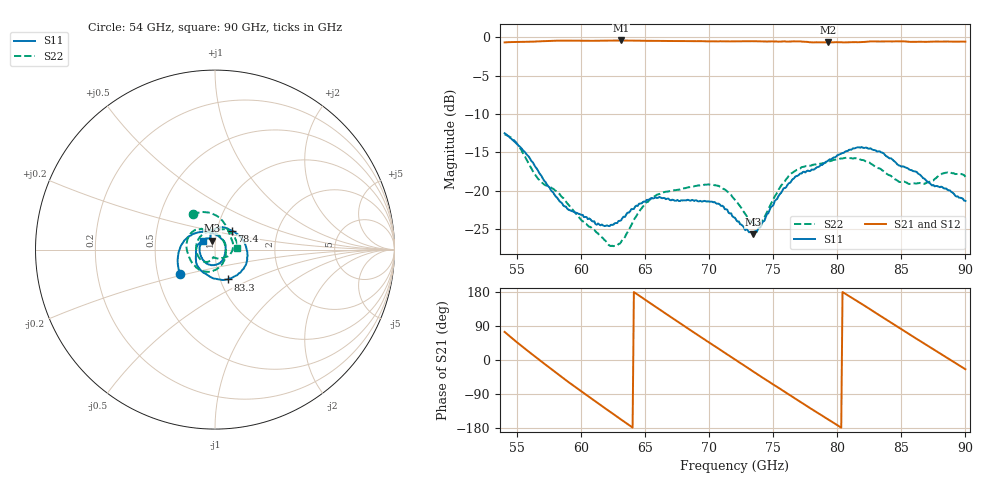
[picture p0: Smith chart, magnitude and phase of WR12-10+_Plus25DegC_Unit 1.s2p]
!Mini-Circuits Laboratory
!S-Parameters
!Model: WR12-10+
!Run / Lot / Date Code: Y97271 / QN2608234 / 2608
!Fixture: N/A, Pressing Arm: N/A
!Network Analyzer: PNA-X N5242B - 423 4 ports (COM/DCOM);  Serial number: 76642
!Date: 3/10/2026 at 2:21:42 PM
!No.: Unit# 1
!Tested with:
# Hz  S  dB  R  50
!Frequency  S11 dB  S11 Deg  S21 dB  S21 Deg  S12 dB  S12 Deg  S22 dB  S22 Deg
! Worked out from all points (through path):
!   352 points, 54 GHz to 90 GHz, reference 50 ohm
!   highest |S21| = -0.41 dB at 63.1 GHz (marker M1); lowest = -0.7 dB at 79.3 GHz (marker M2)
!   lowest |S11| = -25.7 dB at 73.4 GHz (marker M3), VSWR 1.11, Z = 48.4 + j4.85 ohm
!   |S11| at or under -10 dB: start of sweep to end of sweep
!   |S22| runs from -27.3 to -12.7 dB; largest |S21 - S12| = 0.028
!   S11 on the Smith chart (normalised r, x): 54 GHz: 0.65, -0.19; 78.4 GHz: 1.18, +0.26; 83.3 GHz: 1.08, -0.37; 90 GHz: 0.87, +0.09
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5.4e10  -12.52 -145.3  -0.67 74.2  -0.61 74.8  -12.68 122.5
5.55e10  -14.83 166.6  -0.61 32.3  -0.55 32.5  -15.28 78.9
5.69e10  -18.15 126.8  -0.52 -4.5  -0.47 -4.3  -18.94 39.6
5.86e10  -21.97 82.1  -0.43 -48.2  -0.37 -48.2  -20.99 -16.7
6e10  -23.17 45.2  -0.45 -82.9  -0.39 -83.0  -23.87 -46.9
6.14e10  -24.43 7.0  -0.44 -116.4  -0.38 -117.1  -25.82 -75.8
6.31e10  -23.88 -38.0  -0.41 -157.1  -0.37 -157.6  -26.73 -104.5
6.45e10  -21.72 -75.6  -0.44 170.1  -0.39 169.4  -22.79 -116.2
6.6e10  -20.93 -119.1  -0.47 135.8  -0.42 134.8  -20.49 -138.0
6.88e10  -21.35 170.2  -0.50 72.5  -0.44 71.3  -19.45 169.4
7.2e10  -23.55 112.3  -0.53 1.3  -0.48 0.4  -21.21 81.6
7.34e10  -25.68 105.9  -0.51 -29.8  -0.48 -30.2  -24.23 24.1
7.58e10  -19.70 99.2  -0.52 -82.1  -0.62 -82.8  -18.86 -89.5
7.8e10  -17.26 57.7  -0.66 -129.9  -0.61 -129.3  -16.70 -147.5
7.84e10  -16.96 48.5  -0.65 -138.2  -0.60 -138.0  -16.54 -156.5
7.93e10  -16.05 27.4  -0.67 -157.2  -0.60 -157.3  -16.22 -174.6
8.12e10  -14.50 -17.3  -0.63 162.5  -0.64 162.0  -15.81 151.0
8.33e10  -14.87 -67.3  -0.55 117.7  -0.72 118.0  -17.10 124.0
8.4e10  -15.71 -87.2  -0.54 102.7  -0.68 103.3  -17.97 120.1
8.57e10  -17.31 -129.4  -0.60 66.3  -0.58 67.4  -19.12 101.3
8.75e10  -19.27 -168.0  -0.56 28.5  -0.56 29.2  -18.68 75.1
9e10  -21.35 144.2  -0.57 -24.5  -0.48 -23.7  -18.21 4.5
